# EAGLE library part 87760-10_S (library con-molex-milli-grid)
HEADER
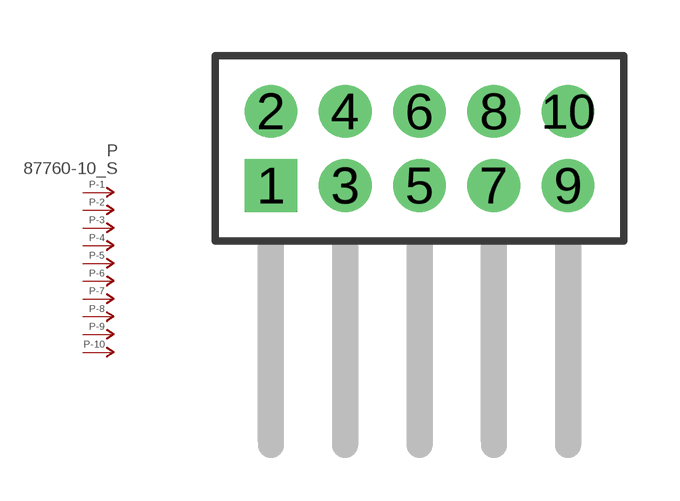
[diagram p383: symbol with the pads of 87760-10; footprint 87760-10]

Designator prefix P; gates -1=P-NV -2=P-N -3=P-N -4=P-N -5=P-N -6=P-N -7=P-N -8=P-N -9=P-N -10=P-N

## 87760-10_S  [87760-10]
1  -1:P  pas
2  -2:P  pas
3  -3:P  pas
4  -4:P  pas
5  -5:P  pas
6  -6:P  pas
7  -7:P  pas
8  -8:P  pas
9  -9:P  pas
10  -10:P  pas

## Footprint 87760-10 (pad centres in mm)
HEADER Dual Row, Right Angle
drill 0.914 square: 1 -4,-1
drill 0.914: 2 -4,1; 3 -2,-1; 4 -2,1; 5 0,-1; 6 0,1; 7 2,-1; 8 2,1; 9 4,-1; 10 4,1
